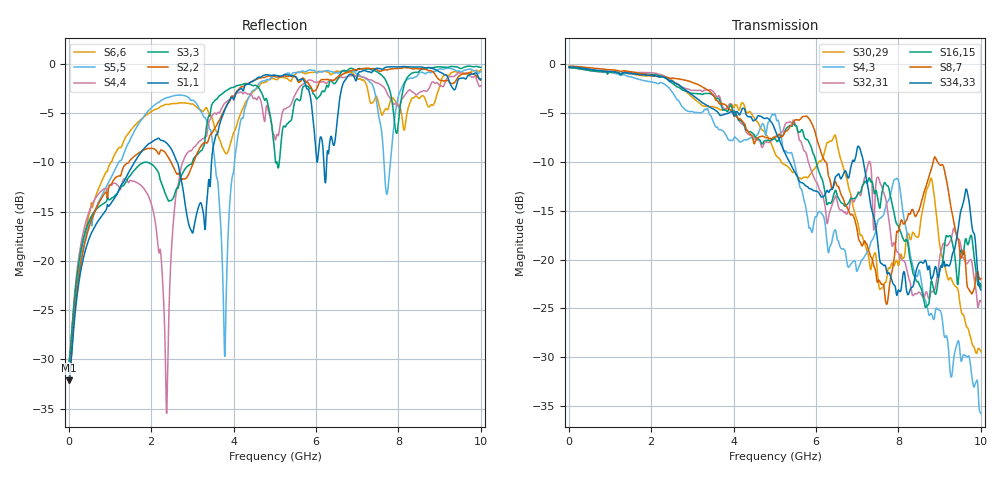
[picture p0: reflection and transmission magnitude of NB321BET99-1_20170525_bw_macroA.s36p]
! Touchstone(R) file created by SIwave 2017.0.0
! Touchstone(R) file created on Fri Jun 02 15:57:50 2017
! Port[1] = D_AN_0__DIE_461
! Port[2] = D_AN_0__LGA_F2
! Port[3] = D_AN_1__DIE_457
! Port[4] = D_AN_1__LGA_G1
! Port[5] = D_AN_2__DIE_453
! Port[6] = D_AN_2__LGA_B6
! Port[7] = D_AN_3__DIE_447
! Port[8] = D_AN_3__LGA_L1
! Port[9] = D_AN_4__DIE_437
! Port[10] = D_AN_4__LGA_A7
! Port[11] = D_AN_5__DIE_431
! Port[12] = D_AN_5__LGA_A9
! Port[13] = D_AN_6__DIE_427
! Port[14] = D_AN_6__LGA_T2
! Port[15] = D_AN_7__DIE_423
! Port[16] = D_AN_7__LGA_U1
! Port[17] = D_AP_0__DIE_460
! Port[18] = D_AP_0__LGA_E1
! Port[19] = D_AP_1__DIE_456
! Port[20] = D_AP_1__LGA_J1
! Port[21] = D_AP_2__DIE_452
! Port[22] = D_AP_2__LGA_A5
! Port[23] = D_AP_3__DIE_446
! Port[24] = D_AP_3__LGA_K2
! Port[25] = D_AP_4__DIE_436
! Port[26] = D_AP_4__LGA_B8
! Port[27] = D_AP_5__DIE_430
! Port[28] = D_AP_5__LGA_A11
! Port[29] = D_AP_6__DIE_426
! Port[30] = D_AP_6__LGA_R1
! Port[31] = D_AP_7__DIE_422
! Port[32] = D_AP_7__LGA_W1
! Port[33] = DCLK_AN_DIE_442
! Port[34] = DCLK_AN_LGA_N1
! Port[35] = DCLK_AP_DIE_441
! Port[36] = DCLK_AP_LGA_P2
! S-parameters (magnitude in dB)
# Hz S DB R 50.000000
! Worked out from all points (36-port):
!   1000 points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, 10 MHz to 10 GHz, reference 50 ohm
!   strongest paths, dB at 10 MHz, 2.51 GHz, 5.01 GHz, 7.51 GHz, 10 GHz:
!     S34,33: -0.3, -1.7, -6.8, -18.7, -23.1
!     S8,7: -0.2, -1.4, -7.5, -22.2, -21.9
!     S16,15: -0.4, -1.9, -7.7, -14.1, -22.8
!     S32,31: -0.4, -1.7, -7.4, -11.6, -24.3
!     S4,3: -0.3, -2.9, -5.1, -15.9, -35.7
!     S30,29: -0.3, -1.7, -9.2, -22.2, -29.4
!   lowest |S11| = -32.1 dB at 10 MHz (marker M1), VSWR 1.05, Z = 52.5 + j0.309 ohm
!   |S11| at or under -10 dB: start of sweep to 1.595 GHz; 2.635 GHz to 3.465 GHz (830.2 MHz wide, 27.2 % of centre); 6.189 GHz to 6.257 GHz (67.59 MHz wide, 1.09 % of centre)
